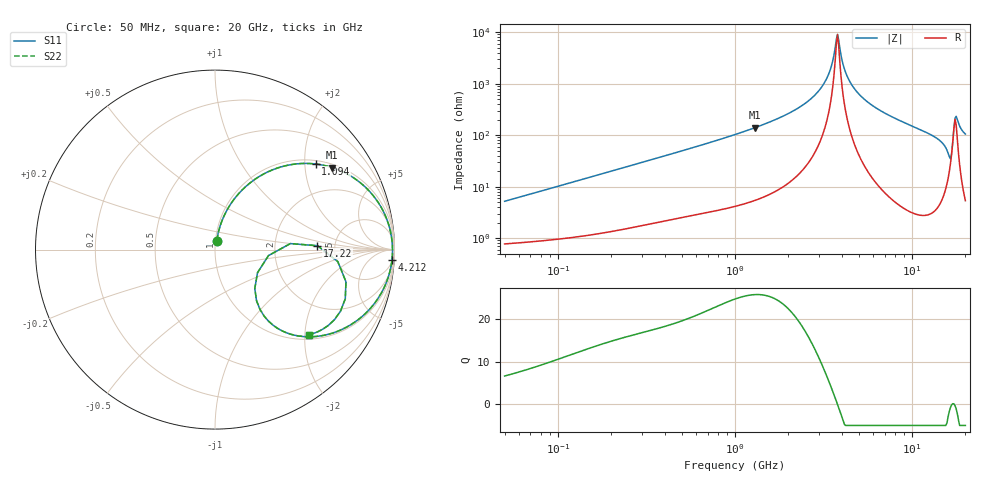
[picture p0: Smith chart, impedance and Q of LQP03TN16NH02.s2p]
!Murata Part Number: LQP03TN16NH02
!These Parameters are Measured in Series Mode Connection
!  o--[Z]--o
!Port1  Port2
!  o-------o
!Freq. Start=50[MHz] Stop=20[GHz], 401[Steps]
# Hz S RI R 50
!Freq.(Hz) S11(Real) S11(Imag) S21(Real) S21(Imag) S12(Real) S12(Imag) S22(Real) S22(Imag)
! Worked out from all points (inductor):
!   401 points, 50 MHz to 20 GHz, reference 50 ohm
!   read as one part in series: L = 16.2 nH near 51.52 MHz
!   highest Q = 25.9 at 1.29 GHz (marker M1), where L = 17.1 nH
!   self-resonance near 3.736 GHz
!   S11 on the Smith chart (normalised r, x): 50 MHz: 1.02, +0.10; 1.094 GHz: 1.09, +2.27; 4.212 GHz: 7, -33; 17.22 GHz: 3.65, +0.24; 20 GHz: 1.11, -2.09
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5e7  0.0102 0.0504  0.9898 -0.0504  0.9898 -0.0504  0.0102 0.0504
1.364002e8  0.0286 0.1315  0.9714 -0.1315  0.9714 -0.1315  0.0286 0.1315
3.721004e8  0.1322 0.312  0.8678 -0.312  0.8678 -0.312  0.1322 0.312
1e9  0.512 0.4801  0.488 -0.4801  0.488 -0.4801  0.512 0.4801
1.094034e9  0.5614 0.4769  0.4386 -0.4769  0.4386 -0.4769  0.5614 0.4769
1.289994e9  0.6523 0.4573  0.3477 -0.4573  0.3477 -0.4573  0.6523 0.4573
1.99176e9  0.8608 0.3247  0.1392 -0.3247  0.1392 -0.3247  0.8608 0.3247
2.728004e9  0.9545 0.1761  0.0455 -0.1761  0.0455 -0.1761  0.9545 0.1761
3.314454e9  0.983 0.0731  0.017 -0.0731  0.017 -0.0731  0.983 0.0731
3.792786e9  0.989 -0.000452  0.011 0.000452  0.011 0.000452  0.989 -0.000452
4.212059e9  0.986 -0.058  0.014 0.058  0.014 0.058  0.986 -0.058
4.539627e9  0.9796 -0.0989  0.0204 0.0989  0.0204 0.0989  0.9796 -0.0989
5.117541e9  0.9619 -0.1636  0.0381 0.1636  0.0381 0.1636  0.9619 -0.1636
7.442007e9  0.846 -0.3483  0.154 0.3483  0.154 0.3483  0.846 -0.3483
1.396067e10  0.4195 -0.4707  0.5805 0.4707  0.5805 0.4707  0.4195 -0.4707
1.527346e10  0.2988 -0.3993  0.7012 0.3993  0.7012 0.3993  0.2988 -0.3993
1.621653e10  0.2218 -0.2161  0.7782 0.2161  0.7782 0.2161  0.2218 -0.2161
1.670968e10  0.2983 -0.033  0.7017 0.033  0.7017 0.033  0.2983 -0.033
1.721783e10  0.571 0.0218  0.429 -0.0218  0.429 -0.0218  0.571 0.0218
1.800918e10  0.7258 -0.2745  0.2742 0.2745  0.2742 0.2745  0.7258 -0.2745
1.88369e10  0.6317 -0.4222  0.3683 0.4222  0.3683 0.4222  0.6317 -0.4222
2e10  0.5225 -0.4747  0.4775 0.4747  0.4775 0.4747  0.5225 -0.4747
